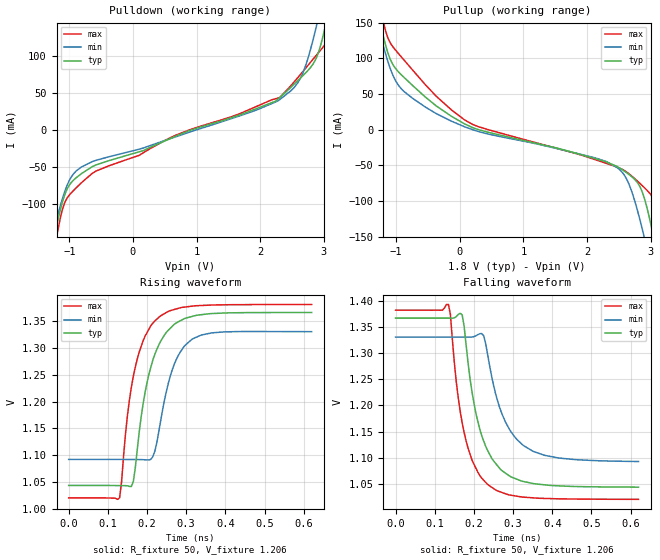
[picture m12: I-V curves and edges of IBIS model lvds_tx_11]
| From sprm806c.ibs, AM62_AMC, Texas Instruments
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|   MODEL lvds_tx_11
[Model] lvds_tx_11
Model_type Output
C_comp 1.664p 1.723p 1.554p
Vmeas = 1.2
Vref = 1.2V
Rref = 50
Cref = 0.5pF
[Model Spec]
[Temperature Range]  40 150 -40
[Voltage Range] 1.8 1.62 1.98
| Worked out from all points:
|   slope of the pulldown table from 0 to 0.27 V, typ, clamps not added: 32.3 ohm
|   slope of the pullup table from 0 to 0.27 V, typ, clamps not added: 24.1 ohm
|   rising waveform, R_fixture 50, V_fixture 1.206: 20-80 % time 52.9ps typ, 48.6ps min, 48.4ps max; typ from 1.04 V to 1.37 V
|   falling waveform, R_fixture 50, V_fixture 1.206: 20-80 % time 56.8ps typ, 65.4ps min, 49.9ps max; typ from 1.37 V to 1.04 V
[Pulldown]
-1.71V    -379.1mA   -326.7mA   -450.1mA
-1.245V   -150.3mA   -138.1mA   -169.3mA
-1.182V   -124mA     -116.1mA   -137.3mA
-1.034V   -80.22mA   -75.15mA   -92.39mA
-807.3mV  -59.2mA    -50.24mA   -71.42mA
670.8mV   -8.691mA   -9.675mA   -7.424mA
2.281V    41.28mA    39.02mA    42.79mA
2.634V    69.86mA    69.7mA     74.69mA
2.883V    96.88mA    139.1mA    100.5mA
3.03V     142.3mA    195.8mA    116.2mA
3.152V    195.4mA    245.4mA    140.7mA
3.511V    373.6mA    396.2mA    335.2mA
[Pullup]
-1.711V   373.6mA    320.4mA    445.7mA
-1.273V   159.8mA    142.8mA    185.2mA
-1.183V   124.5mA    111.8mA    144.7mA
-998.1mV  84.66mA    67.09mA    110.4mA
-538.9mV  45.69mA    31.69mA    62.97mA
203.5mV   2.958mA    0A         7.386mA
2.301V    -45.05mA   -44.57mA   -47.01mA
2.618V    -59.94mA   -68.35mA   -58.95mA
2.882V    -90.67mA   -144.1mA   -79.47mA
3.04V     -148mA     -205.8mA   -96.57mA
3.183V    -214.2mA   -264.7mA   -147.2mA
3.51V     -379.1mA   -402.9mA   -338.1mA
[Ramp]
dV/dt_r .194/53.17p .143/48.566p .217/48.672p
dV/dt_f .194/56.854p .143/65.683p .217/49.605p
[Rising Waveform]
R_fixture = 50
V_fixture = 1.206
V_fixture_min = 1.212
V_fixture_max = 1.202
0s        1.043V     1.092V     1.02V
130ps     1.043V     1.092V     1.02V
150ps     1.043V     1.092V     1.174V
170ps     1.076V     1.092V     1.265V
200ps     1.236V     1.091V     1.329V
220ps     1.289V     1.108V     1.351V
235ps     1.313V     1.165V     1.361V
270ps     1.345V     1.271V     1.373V
315ps     1.359V     1.317V     1.379V
620ps     1.367V     1.331V     1.382V
[Falling Waveform]
R_fixture = 50
V_fixture = 1.206
V_fixture_min = 1.212
V_fixture_max = 1.202
0s        1.367V     1.331V     1.383V
135ps     1.367V     1.331V     1.393V
155ps     1.37V      1.331V     1.245V
175ps     1.352V     1.331V     1.149V
205ps     1.185V     1.334V     1.08V
225ps     1.132V     1.334V     1.056V
235ps     1.114V     1.298V     1.049V
270ps     1.076V     1.187V     1.034V
325ps     1.054V     1.124V     1.024V
620ps     1.043V     1.093V     1.02V
